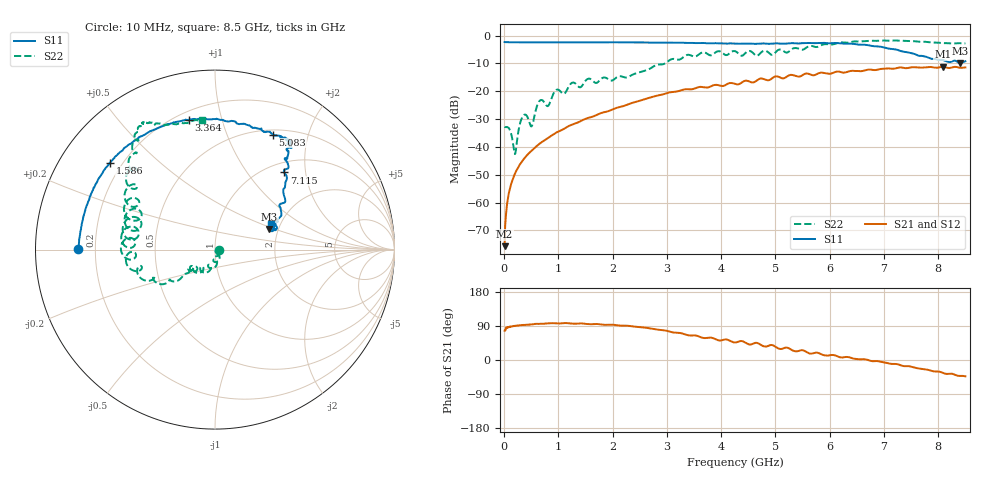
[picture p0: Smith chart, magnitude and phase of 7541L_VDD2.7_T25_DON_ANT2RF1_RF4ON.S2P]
!Agilent Technologies,E5071C,MY46417908,A.11.23
!Date: Wed Dec 09 17:18:17 2020
!Data & Calibration Information:
!Freq	S11:SOLT2(ON)	S21:SOLT2(ON)	S12:SOLT2(ON)	S22:SOLT2(ON)
!PortZ  Port1:50+j0  Port2:50+j0
!Above PortZ is port z conversion or system Z0 setting when saving the data.
!When reading, reference impedance value at option line is always used.
# Hz S dB R 50
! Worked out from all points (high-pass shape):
!   1601 points, 10 MHz to 8.5 GHz, reference 50 ohm
!   highest |S21| = -11.20 dB at 8.081 GHz (marker M1); lowest = -75.6 dB at 10 MHz (marker M2)
!   |S21| within 3 dB of the highest: 5.5 GHz to 5.674 GHz (173.9 MHz wide, 3.11 % of centre); 5.722 GHz to end of sweep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
!   lowest |S11| = -9.8 dB at 8.41 GHz (marker M3), VSWR 1.95, Z = 89.4 + j23.1 ohm
!   |S11| at or under -10 dB: nowhere
!   |S22| runs from -42.6 to -1.8 dB; largest |S21 - S12| = 0.0029
!   S11 on the Smith chart (normalised r, x): 10 MHz: 0.13, +0.00; 1.586 GHz: 0.15, +0.35; 3.364 GHz: 0.25, +0.79; 5.083 GHz: 0.56, +1.48; 7.115 GHz: 1.19, +1.53; 8.5 GHz: 1.80, +0.58
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1e7  -2.34 179.6  -75.64 77.1  -74.35 84.6  -32.76 -7.0
8.42875e7  -2.39 177.6  -56.96 87.5  -56.88 86.9  -33.19 -48.8
2.01025e8  -2.42 174.3  -49.58 90.2  -49.56 90.2  -42.58 -46.6
3.124562e8  -2.44 171.2  -45.69 91.8  -45.66 91.7  -30.41 -40.8
3.9205e8  -2.43 169.1  -43.64 92.7  -43.66 92.8  -28.40 -76.4
5.087875e8  -2.44 166.1  -41.35 94.0  -41.33 94.3  -32.60 -72.9
6.4675e8  -2.43 162.6  -38.96 95.4  -38.97 95.5  -23.65 -74.7
8.112438e8  -2.44 158.5  -36.76 96.8  -36.78 96.8  -25.28 -89.6
9.65125e8  -2.41 154.7  -34.81 96.7  -34.83 96.6  -19.51 -99.5
1.426769e9  -2.38 143.9  -30.56 96.5  -30.57 96.5  -18.30 -121.8
1.585956e9  -2.39 140.4  -29.39 94.3  -29.40 94.3  -15.56 -136.4
2.265156e9  -2.46 125.3  -24.86 90.5  -24.85 90.5  -15.04 -141.2
2.843538e9  -2.53 112.5  -21.51 79.8  -21.52 79.8  -10.41 -145.3
3.36355e9  -2.64 101.4  -19.25 66.2  -19.26 66.2  -7.01 -159.7
4.255e9  -2.84 80.8  -17.37 46.3  -17.37 46.2  -5.61 169.4
5.082775e9  -2.88 63.2  -15.02 29.2  -14.98 29.1  -5.01 153.0
5.671769e9  -2.73 57.0  -14.19 17.0  -14.13 16.9  -3.73 135.8
7.088538e9  -4.69 48.8  -11.79 -9.1  -11.85 -9.1  -1.85 119.7
7.115069e9  -4.77 48.1  -11.84 -9.8  -11.88 -9.7  -1.84 119.8
8.080806e9  -8.75 19.0  -11.20 -33.5  -11.23 -33.5  -2.69 107.8
8.409794e9  -9.81 20.9  -11.58 -42.0  -11.63 -42.2  -2.75 98.2
8.5e9  -9.24 24.3  -11.46 -43.1  -11.54 -43.0  -2.82 95.8
